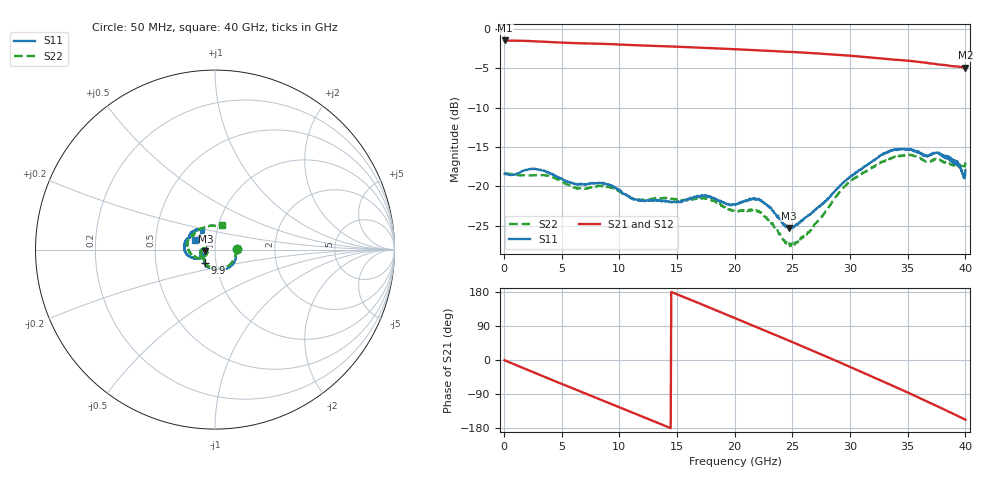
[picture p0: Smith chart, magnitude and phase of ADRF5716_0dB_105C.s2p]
! Device: ADRF5716
! Description: 30GHz 2-Bit Digital Attenuator
! Frequency: 100 MHz – 30 GHz
! Ports:
! ATTIN  = Port 1
! ATTOUT = Port 2
! State: 0 dB Attenuation selected
! Supply Voltage:
! VDD  =  +3.30 Volts
! VSS  =  -3.30 Volts
! Control Voltages:
! D5 = 0V, D6 = 0V
! Temperature = +105 C
! Data: Data was collected using a calibrated network analyzer.
!  The reference plane is the package pins of ADRF5716 switch.
! Note: Analog Devices supplies this data as a sample of measured data for this product.
!  Your particular data for this product may vary.
!  Analog Devices reserves the right to change this data at anytime
# HZ S DB R 50
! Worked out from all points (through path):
!   800 points, 50 MHz to 40 GHz, reference 50 ohm
!   highest |S21| = -1.47 dB at 100 MHz (marker M1); lowest = -4.9 dB at 40 GHz (marker M2)
!   group delay of S21, straight-line fit = 35.5 ps
!   lowest |S11| = -25.3 dB at 24.7 GHz (marker M3), VSWR 1.12, Z = 44.9 - j0.842 ohm
!   |S11| at or under -10 dB: start of sweep to end of sweep
!   |S22| runs from -27.6 to -16.0 dB; largest |S21 - S12| = 0
!   S11 on the Smith chart (normalised r, x): 50 MHz: 1.27, +0.01; 9.9 GHz: 0.88, -0.14; 40 GHz: 0.79, +0.09
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5e7  -18.40 1.1  -1.47 -0.6  -1.47 -0.6  -18.34 1.8
1e8  -18.38 -1.5  -1.47 -1.4  -1.47 -1.4  -18.32 -1.6
1.8e9  -17.94 -25.2  -1.52 -23.0  -1.52 -23.0  -18.62 -27.2
3.75e9  -18.16 -59.9  -1.66 -47.6  -1.66 -47.6  -18.66 -56.3
6.75e9  -19.71 -93.2  -1.83 -84.6  -1.83 -84.6  -20.29 -90.5
8.3e9  -19.56 -109.1  -1.89 -103.8  -1.89 -103.8  -19.92 -105.1
9.9e9  -20.39 -127.1  -1.98 -123.5  -1.98 -123.5  -20.53 -123.9
1.17e10  -21.76 -134.4  -2.09 -145.6  -2.09 -145.6  -21.66 -132.9
1.34e10  -21.79 -141.2  -2.18 -166.7  -2.18 -166.7  -21.43 -141.9
1.49e10  -22.00 -146.1  -2.26 174.6  -2.26 174.6  -21.63 -151.3
1.655e10  -21.34 -151.4  -2.36 154.3  -2.36 154.3  -21.59 -158.3
2.005e10  -22.26 -164.1  -2.59 110.3  -2.59 110.3  -23.15 -175.1
2.21e10  -21.57 -173.8  -2.73 84.4  -2.73 84.4  -23.12 176.8
2.47e10  -25.28 -170.1  -2.92 51.1  -2.92 51.1  -27.33 -174.7
2.67e10  -23.36 -153.0  -3.08 25.2  -3.08 25.2  -25.34 -149.7
2.83e10  -21.20 -148.9  -3.24 4.3  -3.24 4.3  -22.39 -145.6
2.99e10  -18.93 -153.1  -3.40 -16.8  -3.40 -16.8  -19.47 -153.6
3.335e10  -15.59 -176.1  -3.85 -63.3  -3.85 -63.3  -16.66 -179.9
3.495e10  -15.27 167.2  -4.03 -85.0  -4.03 -85.0  -16.03 162.9
3.64e10  -16.10 154.5  -4.28 -105.4  -4.28 -105.4  -16.71 147.1
3.77e10  -15.73 143.3  -4.53 -124.0  -4.53 -124.0  -16.61 134.0
4e10  -17.98 154.4  -4.93 -157.6  -4.93 -157.6  -16.96 73.8
